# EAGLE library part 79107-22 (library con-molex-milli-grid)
RECEPTACAL
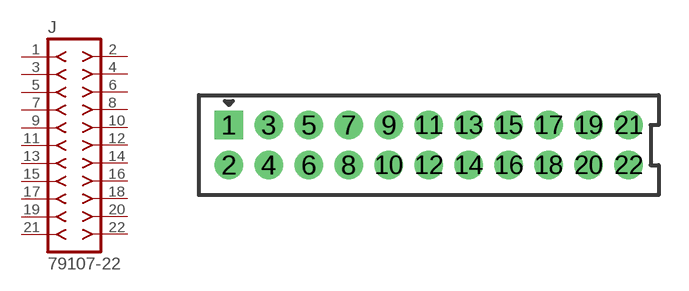
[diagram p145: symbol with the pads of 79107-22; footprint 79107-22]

Designator prefix J

## 79107-22  [79107-22]
1  1  pas
2  2  pas
3  3  pas
4  4  pas
5  5  pas
6  6  pas
7  7  pas
8  8  pas
9  9  pas
10  10  pas
11  11  pas
12  12  pas
13  13  pas
14  14  pas
15  15  pas
16  16  pas
17  17  pas
18  18  pas
19  19  pas
20  20  pas
21  21  pas
22  22  pas

## Footprint 79107-22 (pad centres in mm)
RECEPTACAL Dual Row, Vertical, Through-Hole
drill 0.914 square: 1 -10,1
drill 0.914: 2 -10,-1; 3 -8,1; 4 -8,-1; 5 -6,1; 6 -6,-1; 7 -4,1; 8 -4,-1; 9 -2,1; 10 -2,-1; 11 0,1; 12 0,-1; 13 2,1; 14 2,-1; 15 4,1; 16 4,-1; 17 6,1; 18 6,-1; 19 8,1; 20 8,-1; 21 10,1; 22 10,-1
